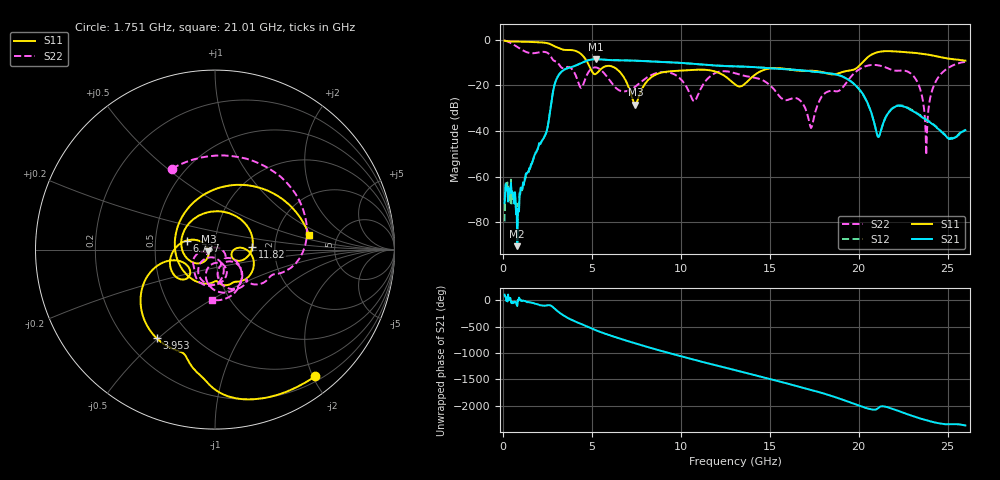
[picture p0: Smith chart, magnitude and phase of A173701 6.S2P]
!  2-Port S-parameters saved by WinCal
! VAR MeasName=S-Parameters (CALIBRATED_DATA) read from VNA (N5245A)
! VAR MeasDate=2017-6-7 10:28:48
! VAR NAME=A173701 6
! VAR FILENAME=A173701 6.S2P
! VAR DATE=2017-6-7 10:28:48
! VAR PHYS_PORTS=1,2
# Hz S DB R 50
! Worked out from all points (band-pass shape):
!   801 points, 100 MHz to 26 GHz, reference 50 ohm
!   highest |S21| = -8.46 dB at 5.248 GHz (marker M1); lowest = -90.5 dB at 812.2 MHz (marker M2)
!   |S21| within 3 dB of the highest: 4.034 GHz to 12.44 GHz (8.406 GHz wide, 102 % of centre)
!   lowest |S11| = -28.5 dB at 7.449 GHz (marker M3), VSWR 1.08, Z = 46.5 - j0.88 ohm
!   |S11| at or under -10 dB: 4.763 GHz to 20.2 GHz (15.44 GHz wide, 124 % of centre)
!   |S22| runs from -50.5 to -0.2 dB; largest |S21 - S12| = 0.0046
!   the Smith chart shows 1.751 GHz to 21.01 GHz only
!   S11 on the Smith chart (normalised r, x): 1.751 GHz: 0.28, -2.04; 3.953 GHz: 0.33, -0.49; 6.737 GHz: 0.72, +0.08; 11.82 GHz: 1.52, +0.04; 21.01 GHz: 3.08, +0.70
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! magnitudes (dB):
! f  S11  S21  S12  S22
! 100 MHz  -0.3  -71.7  -79.7  -0.2
! 261.9 MHz  -0.6  -65.1  -62.6  -0.7
! 812.2 MHz  -0.8  -90.5  -82.5  -3.1
! 1.751 GHz  -0.9  -51.5  -51.1  -5.8
! 3.046 GHz  -3.2  -16.7  -16.7  -9.7
! 3.953 GHz  -4.6  -11.7  -11.6  -13.5
! 4.438 GHz  -6.5  -10.1  -10.0  -20.9
! 5.248 GHz  -14.9  -8.5  -8.5  -12.1
! 6.737 GHz  -15.6  -9.0  -9.0  -22.6
! 7.449 GHz  -28.5  -9.1  -9.1  -20.5
! 8.744 GHz  -14.8  -9.6  -9.6  -14.4
! 10.75 GHz  -13.1  -10.5  -10.5  -27.0
! 11.82 GHz  -13.6  -11.2  -11.2  -15.1
! 13.05 GHz  -19.5  -11.6  -11.6  -14.6
! 17.39 GHz  -13.5  -13.9  -13.8  -37.6
! 19.78 GHz  -12.8  -19.6  -19.7  -14.4
! 21.01 GHz  -5.5  -40.9  -40.9  -11.1
! 21.69 GHz  -4.9  -31.9  -31.7  -12.7
! 23.18 GHz  -5.7  -31.9  -31.6  -16.9
! 23.8 GHz  -6.3  -35.1  -34.9  -50.5
! 24.45 GHz  -7.3  -38.9  -38.7  -16.8
! 26 GHz  -9.1  -39.6  -39.6  -9.7
